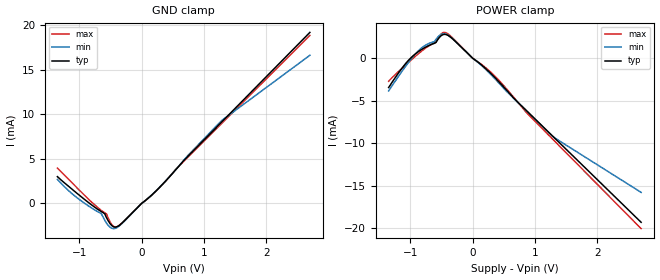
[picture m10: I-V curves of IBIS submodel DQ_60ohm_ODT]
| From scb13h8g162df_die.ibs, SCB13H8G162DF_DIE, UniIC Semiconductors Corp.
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|   Submodel DQ_60ohm_ODT
[Submodel] DQ_60ohm_ODT
Submodel_type Dynamic_clamp
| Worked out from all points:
|   GND clamp passes 1 mA (typ) near -0.14 V on its own axis
|   POWER clamp passes 1 mA (typ) near -0.14 V on its own axis
[GND_clamp]
|Voltage   I(typ)   I(min)   I(max)
-1.35V    3.006mA    2.698mA    3.965mA
-1.041V   1.167mA    670.2uA    1.787mA
-647mV    -908.7uA   -1.132mA   -773.6uA
-591mV    -1.159mA   -1.876mA   -1.054mA
-563mV    -1.586mA   -2.199mA   -1.174mA
-506mV    -2.262mA   -2.662mA   -2.061mA
-450mV    -2.618mA   -2.828mA   -2.572mA
-394mV    -2.612mA   -2.706mA   -2.605mA
253mV     1.545mA    1.562mA    1.527mA
562mV     3.887mA    3.913mA    3.927mA
1.294V    9.193mA    9.344mA    9.032mA
2.7V      19.18mA    16.62mA    18.85mA
[POWER_clamp]
|Voltage   I(typ)   I(min)   I(max)
-1.35V    -3.429mA   -3.828mA   -2.692mA
-1.069V   -536.4uA   -840.9uA   -723.5uA
-844mV    938.9uA    1.085mA    717.9uA
-591mV    1.875mA    2.229mA    1.887mA
-534mV    2.478mA    2.696mA    2.648mA
-478mV    2.792mA    2.891mA    3.027mA
-394mV    2.69mA     2.704mA    2.857mA
100nV     -189nA     -184.7nA   -197nA
338mV     -2.136mA   -2.27mA    -1.972mA
872mV     -6.226mA   -6.253mA   -6.467mA
1.294V    -9.239mA   -9.257mA   -9.597mA
2.7V      -19.28mA   -15.76mA   -20.03mA
